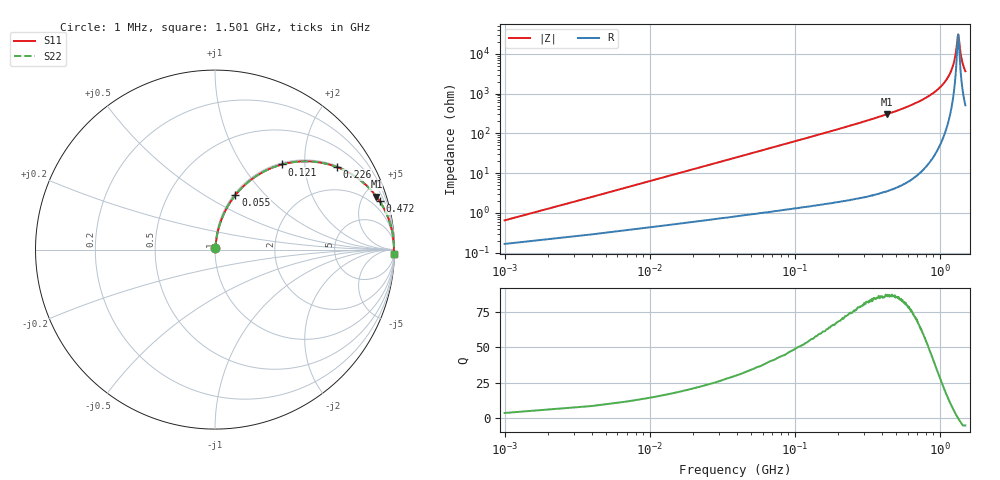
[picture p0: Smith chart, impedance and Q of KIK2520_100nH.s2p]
!version-2
!date-01.2022
!Series
# MHz S RI R 50
!Freq ReS11 ImS11 ReS21 ImS21 ReS12 ImS12 ReS22 ImS22
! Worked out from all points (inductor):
!   501 points, 1 MHz to 1.501 GHz, reference 50 ohm
!   read as one part in series: L = 100 nH near 7 MHz
!   highest Q = 86.6 at 433 MHz (marker M1), where L = 112 nH
!   self-resonance near 1.336 GHz
!   S11 on the Smith chart (normalised r, x): 1 MHz: 1.00, +0.01; 55 MHz: 1.02, +0.69; 121 MHz: 1.03, +1.53; 226 MHz: 1.04, +2.92; 472 MHz: 1.08, +6.77; 1.501 GHz: 11, -72
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1  0.0017 0.00626  0.9983 -0.00626  0.9983 -0.00626  0.0017 0.00626
10  0.0082 0.0621  0.9918 -0.0621  0.9918 -0.0621  0.0082 0.0621
16  0.0152 0.0985  0.9848 -0.0985  0.9848 -0.0985  0.0152 0.0985
31  0.0431 0.1851  0.9569 -0.1851  0.9569 -0.1851  0.0431 0.1851
55  0.1137 0.3039  0.8863 -0.3039  0.8863 -0.3039  0.1137 0.3039
121  0.3725 0.4742  0.6275 -0.4742  0.6275 -0.4742  0.3725 0.4742
226  0.6789 0.46  0.3211 -0.46  0.3211 -0.46  0.6789 0.46
253  0.7284 0.4382  0.2716 -0.4382  0.2716 -0.4382  0.7284 0.4382
433  0.8995 0.2949  0.1005 -0.2949  0.1005 -0.2949  0.8995 0.2949
472  0.9172 0.2699  0.0828 -0.2699  0.0828 -0.2699  0.9172 0.2699
502  0.9284 0.2521  0.0716 -0.2521  0.0716 -0.2521  0.9284 0.2521
751  0.9771 0.1415  0.0228 -0.1415  0.0228 -0.1415  0.9771 0.1415
1003  0.9928 0.0689  0.00723 -0.0689  0.00723 -0.0689  0.9928 0.0689
1153  0.996 0.0354  0.00399 -0.0354  0.00399 -0.0354  0.996 0.0354
1252  0.9968 0.0158  0.00323 -0.0158  0.00323 -0.0158  0.9968 0.0158
1288  0.9968 0.00911  0.00317 -0.00911  0.00317 -0.00911  0.9968 0.00911
1330  0.9968 0.00153  0.00321 -0.00153  0.00321 -0.00153  0.9968 0.00153
1339  0.9968 -6.74e-05  0.00324 6.74e-05  0.00324 6.74e-05  0.9968 -6.74e-05
1381  0.9966 -0.00736  0.00343 0.00736  0.00343 0.00736  0.9966 -0.00736
1408  0.9964 -0.0119  0.00361 0.0119  0.00361 0.0119  0.9964 -0.0119
1450  0.996 -0.0189  0.00397 0.0189  0.00397 0.0189  0.996 -0.0189
1501  0.9955 -0.0269  0.00453 0.0269  0.00453 0.0269  0.9955 -0.0269
